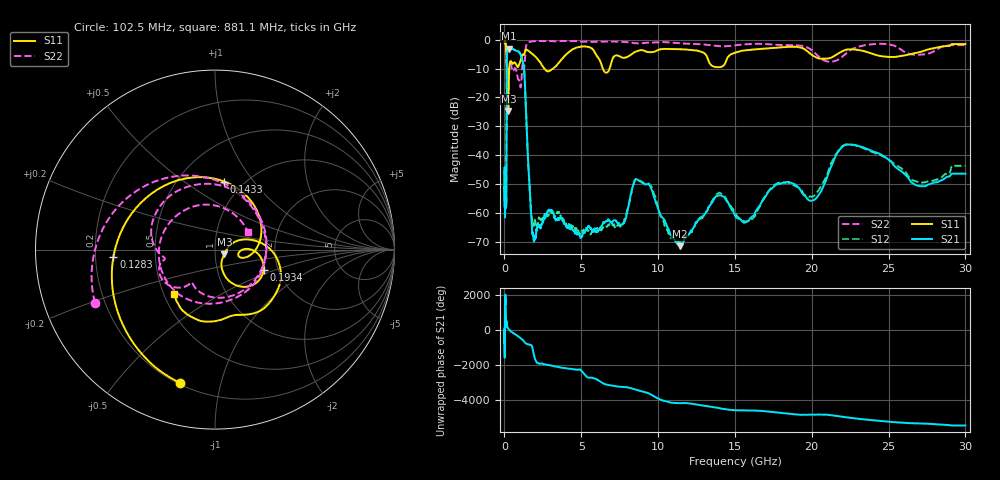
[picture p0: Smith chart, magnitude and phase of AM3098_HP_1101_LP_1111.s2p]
! Date/Time: Thu, Feb 28, 2019 8:46 AM
! Network Analyzer: Agilent Technologies E8364B Rev: A.07.50.67
! Sweep from 0.010 to 30.000 GHz, 1601 Points, Sweep Type: LOG
! Power Supply: 5.023 V, 0.002 A
# Hz S DB R 50
!freq MagS11 AngS11 MagS21 AngS21 MagS12 AngS12 MagS22 AngS22
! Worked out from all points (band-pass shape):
!   1601 points, 10 MHz to 30 GHz, reference 50 ohm
!   highest |S21| = -3.16 dB at 266.5 MHz (marker M1); lowest = -71.4 dB at 11.42 GHz (marker M2)
!   |S21| within 3 dB of the highest: 159.3 MHz to 1.114 GHz (954.7 MHz wide, 150 % of centre)
!   lowest |S11| = -24.7 dB at 252.2 MHz (marker M3), VSWR 1.12, Z = 55.4 - j2.87 ohm
!   |S11| at or under -10 dB: 148 MHz to 314.5 MHz (166.5 MHz wide, 72 % of centre); 2.599 GHz to 3.169 GHz (569.8 MHz wide, 19.8 % of centre); 6.396 GHz to 6.844 GHz (448.2 MHz wide, 6.77 % of centre)
!   |S22| runs from -16.5 to -0.5 dB; largest |S21 - S12| = 0.01
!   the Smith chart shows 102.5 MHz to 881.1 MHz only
!   S11 on the Smith chart (normalised r, x): 102.5 MHz: 0.21, -0.75; 128.3 MHz: 0.28, -0.03; 143.3 MHz: 0.82, +0.73; 193.4 MHz: 1.68, -0.41; 881.1 MHz: 0.57, -0.31
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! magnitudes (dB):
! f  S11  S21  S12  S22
! 10 MHz  -0.4  -46.1  -47.3  -0.6
! 38.04 MHz  -0.3  -57.3  -56.4  -0.9
! 102.5 MHz  -2.3  -57.3  -54.9  -2.7
! 117.9 MHz  -3.5  -55.7  -55.9  -4.1
! 128.3 MHz  -4.9  -39.9  -39.6  -6.3
! 143.3 MHz  -8.3  -15.9  -15.9  -11.0
! 144.7 MHz  -8.8  -14.3  -14.3  -11.1
! 193.4 MHz  -10.7  -4.0  -4.0  -9.7
! 252.2 MHz  -24.7  -3.2  -3.1  -10.9
! 266.5 MHz  -20.0  -3.2  -3.1  -10.8
! 550.5 MHz  -8.3  -3.4  -3.3  -10.9
! 881.1 MHz  -9.5  -4.0  -4.0  -13.6
! 1.27 GHz  -5.3  -9.7  -9.7  -9.9
! 1.758 GHz  -4.7  -61.8  -61.0  -0.6
! 2.084 GHz  -6.3  -65.6  -63.9  -0.5
! 7.926 GHz  -6.1  -61.4  -60.6  -0.9
! 9.118 GHz  -3.9  -49.8  -50.1  -1.1
! 11.42 GHz  -3.3  -71.4  -70.1  -1.3
! 13.88 GHz  -9.6  -54.1  -53.3  -2.2
! 20.1 GHz  -5.6  -55.6  -54.1  -4.1
! 22.56 GHz  -3.4  -36.3  -36.3  -3.5
! 30 GHz  -1.6  -46.4  -43.6  -1.9
